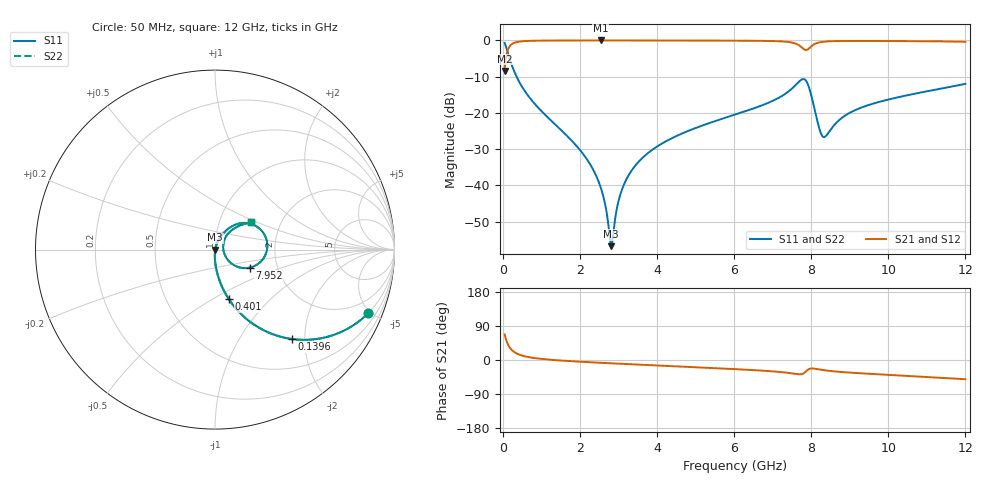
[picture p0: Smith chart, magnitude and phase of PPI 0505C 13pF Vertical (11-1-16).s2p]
# GHz S MA R 50
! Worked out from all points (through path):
!   1601 points, 50 MHz to 12 GHz, reference 50 ohm
!   highest |S21| = -0.01 dB at 2.537 GHz (marker M1); lowest = -8.4 dB at 50 MHz (marker M2)
!   group delay of S21, straight-line fit = 13.8 ps
!   lowest |S11| = -56.8 dB at 2.813 GHz (marker M3), VSWR 1.00, Z = 50.1 - j0.034 ohm
!   |S11| at or under -10 dB: 360 MHz to end of sweep
!   |S22| runs from -56.8 to -0.7 dB; largest |S21 - S12| = 0
!   S11 on the Smith chart (normalised r, x): 50 MHz: 0.99, -4.85; 139.6 MHz: 0.99, -1.73; 401 MHz: 0.99, -0.59; 7.952 GHz: 1.44, -0.30; 12 GHz: 1.41, +0.46
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0.05  0.9252 -22.5  0.3794 67.5  0.3794 67.5  0.9252 -22.5
0.139625  0.6569 -49.3  0.7537 40.6  0.7537 40.6  0.6569 -49.3
0.2441875  0.4441 -64.3  0.8955 25.6  0.8955 25.6  0.4441 -64.3
0.4010313  0.2857 -74.5  0.9577 15.3  0.9577 15.3  0.2857 -74.5
0.9313125  0.1164 -85.8  0.9923 3.8  0.9923 3.8  0.1164 -85.8
2.044156  0.02894 -92.3  0.9982 -4.7  0.9982 -4.7  0.02894 -92.3
2.537094  0.009526 -89.1  0.9984 -7.4  0.9984 -7.4  0.009526 -89.1
2.813438  0.001447 -13.5  0.9984 -8.8  0.9984 -8.8  0.001447 -13.5
3.015094  0.006384 66.7  0.9983 -9.8  0.9983 -9.8  0.006384 66.7
3.209281  0.01213 72.0  0.9982 -10.7  0.9982 -10.7  0.01213 72.0
3.545375  0.02171 73.4  0.9979 -12.3  0.9979 -12.3  0.02171 73.4
4.038312  0.03524 72.5  0.9973 -14.6  0.9973 -14.6  0.03524 72.5
6.025  0.09461 64.0  0.9919 -24.1  0.9919 -24.1  0.09461 64.0
7.585969  0.2384 37.8  0.9086 -36.6  0.9086 -36.6  0.2384 37.8
7.810031  0.2926 5.0  0.7568 -34.8  0.7568 -34.8  0.2926 5.0
7.951937  0.2174 -27.6  0.7825 -23.5  0.7825 -23.5  0.2174 -27.6
8.019156  0.161 -37.0  0.8429 -22.3  0.8429 -22.3  0.161 -37.0
8.220812  0.05836 -24.9  0.9411 -25.2  0.9411 -25.2  0.05836 -24.9
8.340312  0.04639 8.0  0.9612 -27.1  0.9612 -27.1  0.04639 8.0
8.967688  0.09795 50.2  0.9831 -33.0  0.9831 -33.0  0.09795 50.2
10.01331  0.1533 48.3  0.981 -39.3  0.981 -39.3  0.1533 48.3
12  0.2513 37.2  0.9581 -50.7  0.9581 -50.7  0.2513 37.2
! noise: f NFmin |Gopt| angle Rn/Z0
0.05  0.000381  0.8658  1.657  0.00061
1.372  0.003809  0.6616  4.627  0.00215
2.701  0.006306  0.6107  8.451  0.002989
4.031  0.008691  0.5864  12.24  0.003797
5.36  0.01165  0.5907  16.02  0.005118
6.682  0.0197  0.6828  20.08  0.01168
8.012  0.122  0.9301  24.6  0.3703
9.341  0.02821  0.6933  28.04  0.01691
10.67  0.02589  0.6352  31.26  0.01244
12  0.03318  0.6756  35.02  0.01801
